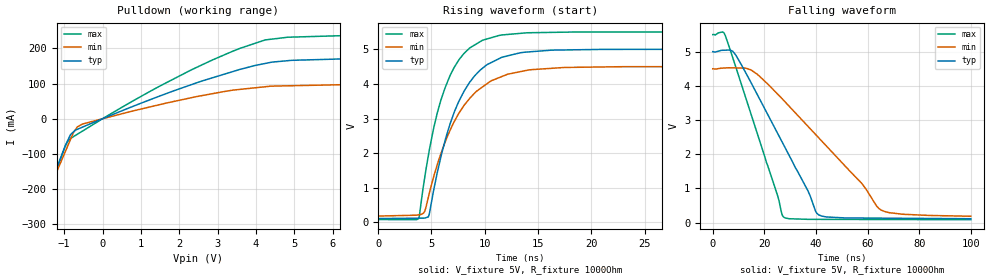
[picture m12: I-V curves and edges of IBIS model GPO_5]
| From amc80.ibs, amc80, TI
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[Model]  GPO_5
Model_type   Open_drain
Polarity   Non-Inverting
Vmeas = 2.5
Vref = 2.5
Cref = 15pF
Rref = 50
|   typ   min   max
|   (nom PVT)   (Fast PVT)   (slow PVT)
|   ON state : BUFFER OUTPUT TURNED HIGH
|C_comp   1.186E-12   9.956E-13   1.413E-12
|   OFF state: BUFFER OUTPUT TURNED LOW
C_comp   9.122E-13   8.552E-13   9.122E-13
| Where   nom PVT is  Nominal Process, 5.0V, 27C
|   Fast PVT is Strong Process, 5.5V, -40C
|   Slow PVT is Weak Process, 4.5V, 125C
|C_comp - from L-C Tank method, L = 1nH, peak frequency
[Voltage Range]   5   4.5   5.5
[Temperature Range]   27   125   -40
[Pullup Reference]   5   4.5   5.5
[Pulldown Reference]   0   0   0
[Power Clamp Reference]   5   4.5   5.5
[GND Clamp Reference]   0   0   0
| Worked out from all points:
|   slope of the pulldown table from 0 to 0.75 V, typ, clamps not added: 22.5 ohm
|   falling waveform, V_fixture 5V, R_fixture 1000Ohm: 20-80 % time 20.4ns typ, 32ns min, 14ns max; typ from 5 V to 0.112 V
|   rising waveform, V_fixture 5V, R_fixture 1000Ohm: 20-80 % time 3.22ns typ, 3.78ns min, 2.73ns max; typ from 0.112 V to 5 V
[Pulldown]
|   Voltage   I(typ)   I(min)   I(max)
-5V       -1.389A    -1.3A      -1.551A
-1.739V   -304.2mA   -303.7mA   -321.7mA
-1.246V   -154.9mA   -164.1mA   -161.1mA
-961.8mV  -74.3mA    -91.31mA   -76.18mA
-836.3mV  -45.18mA   -59.15mA   -56.35mA
-655.4mV  -30.04mA   -23.02mA   -44.02mA
1.48V     64.23mA    39.87mA    92.25mA
3.579V    140.4mA    83.52mA    200.2mA
4.234V    157.2mA    90.98mA    224.1mA
4.826V    165.2mA    93.72mA    232mA
8.622V    174.6mA    99.97mA    242.8mA
9.985V    186.3mA    108.6mA    261.6mA
[Ramp]
R_load = 1000
|   typ   min   max
dV/dt_r   2.9331/3.21982e-009   2.58972/3.77501e-009   3.25004/2.72913e-009
dV/dt_f   2.9331/2.04009e-008   2.58972/3.20414e-008   3.25004/1.39618e-008
[Falling Waveform]
V_fixture = 5V
V_fixture_min = 4.5V
V_fixture_max = 5.5V
R_fixture = 1000Ohm
C_fixture = 0F
|   Time   V(typ)   V(min)   V(max)
0s        5V         4.5V       5.5V
3.755ns   5.04V      4.519V     5.576V
4.832ns   5.043V     4.523V     5.476V
8.823ns   4.911V     4.525V     4.575V
14.79ns   4.101V     4.467V     3.181V
27.54ns   2.262V     3.57V      156mV
41.11ns   222mV      2.474V     92.47mV
57.69ns   131.2mV    1.148V     89.88mV
65.33ns   127.7mV    362mV      88.69mV
100ns     111.5mV    183.8mV    83.27mV
[Rising Waveform]
V_fixture = 5V
V_fixture_min = 4.5V
V_fixture_max = 5.5V
R_fixture = 1000Ohm
C_fixture = 0F
|   Time   V(typ)   V(min)   V(max)
0s        111.5mV    183.8mV    83.26mV
3.799ns   122.9mV    218.4mV    110.1mV
4.36ns    124.5mV    316.2mV    1.282V
4.708ns   160.9mV    723.9mV    1.926V
5.884ns   1.889V     1.98V      3.533V
7.56ns    3.49V      3.147V     4.687V
9.069ns   4.239V     3.737V     5.127V
11.36ns   4.732V     4.183V     5.4V
22.97ns   4.998V     4.497V     5.498V
100ns     5V         4.5V       5.5V
